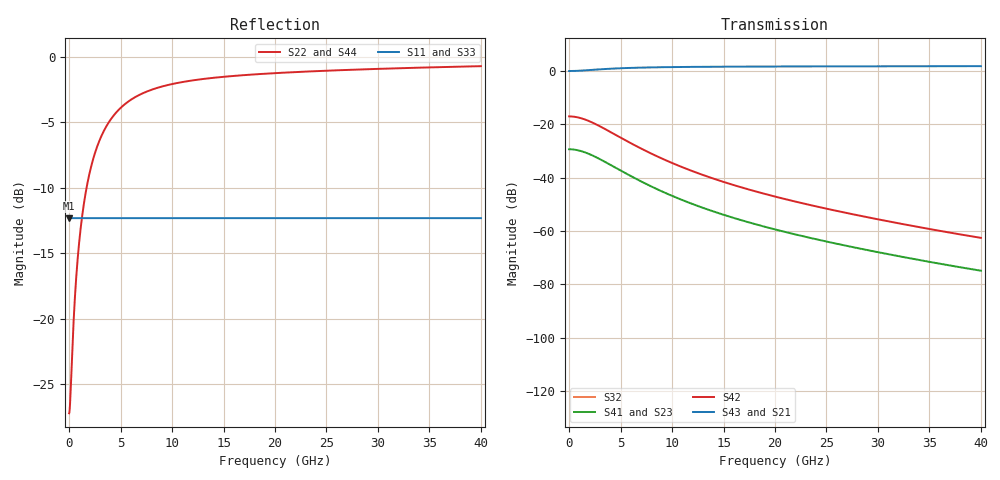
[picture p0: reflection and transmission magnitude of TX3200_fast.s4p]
# hz S ri R 50
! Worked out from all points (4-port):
!   20000 points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, 2 MHz to 40 GHz, reference 50 ohm
!   strongest paths, dB at 2 MHz, 10 GHz, 20 GHz, 30 GHz, 40 GHz:
!     S43: -0.1, 1.4, 1.6, 1.7, 1.7
!     S21: -0.1, 1.4, 1.6, 1.7, 1.7
!     S42: -17.1, -34.5, -47.1, -55.6, -62.6
!     S41: -29.4, -46.8, -59.4, -67.9, -74.9
!     S23: -29.4, -46.8, -59.4, -67.9, -74.9
!     S32: -, -, -, -, -
!   lowest |S11| = -12.3 dB at 2 MHz (marker M1), VSWR 1.64, Z = 82 + j0 ohm
!   |S11| at or under -10 dB: start of sweep to end of sweep
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2000000  0.2426 0  0 0  0 0  0 0
         0.9894 0.000106  0.0436 -0.000437  -0.034 3.53e-05  0.1401 -0.000146
         0 0  0 0  0.2426 0  0 0
         -0.034 3.53e-05  0.1401 -0.000146  0.9905 0.000104  0.0391 -0.00043
7.58e8  0.2426 0  0 0  0 0  0 0
        0.9966 0.0377  0.0139 -0.1555  -0.0304 0.0122  0.1255 -0.0504
        0 0  0 0  0.2426 0  0 0
        -0.0304 0.0122  0.1255 -0.0504  0.9975 0.0373  0.0101 -0.1539
1.64e9  0.2426 0  0 0  0 0  0 0
        1.018 0.0724  -0.0753 -0.2986  -0.0205 0.0209  0.0844 -0.0861
        0 0  0 0  0.2426 0  0 0
        -0.0205 0.0209  0.0844 -0.0861  1.019 0.0718  -0.0774 -0.2961
5.324e9  0.2426 0  0 0  0 0  0 0
         1.117 0.1073  -0.4841 -0.4425  0.00475 0.0116  -0.0196 -0.048
         0 0  0 0  0.2426 0  0 0
         0.00475 0.0116  -0.0196 -0.048  1.117 0.1076  -0.4841 -0.4434
1.009e10  0.2426 0  0 0  0 0  0 0
          1.171 0.0872  -0.703 -0.3593  0.00388 0.00224  -0.016 -0.00924
          0 0  0 0  0.2426 0  0 0
          0.00388 0.00224  -0.016 -0.00924  1.171 0.0875  -0.7056 -0.3609
1.8148e10  0.2426 0  0 0  0 0  0 0
           1.198 0.0635  -0.8179 -0.2617  0.00133 8.01e-05  -0.00548 -0.00033
           0 0  0 0  0.2426 0  0 0
           0.00133 8.05e-05  -0.00548 -0.000332  1.199 0.0633  -0.8214 -0.2608
4e10  0.2426 0  0 0  0 0  0 0
      1.22 0.0412  -0.9065 -0.1698  0.00013 -0.000126  -0.000534 0.000518
      0 0  0 0  0.2426 0  0 0
      0.00013 -0.000125  -0.000536 0.000517  1.22 0.0407  -0.907 -0.1677
